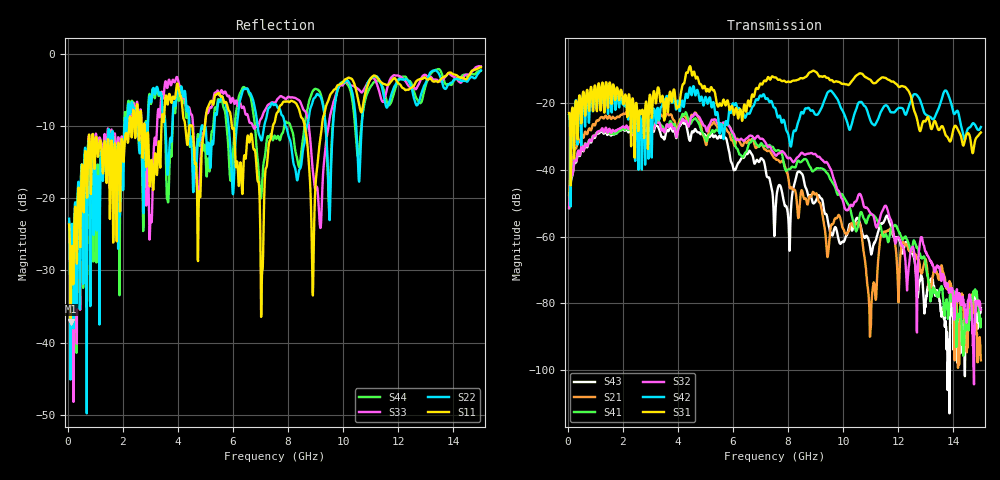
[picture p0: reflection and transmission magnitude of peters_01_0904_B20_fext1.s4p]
# MHZ S RI R 50.00
! FREQ  S11  S12  S13  S14
!  S21  S22  S23  S24
!  S31  S32  S33  S34
!  S41  S42  S43  S44
!  REAL  IMAG  REAL  IMAG  REAL  IMAG  REAL  IMAG
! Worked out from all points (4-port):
!   1496 points, 50 MHz to 15 GHz, reference 50 ohm
!   strongest paths, dB at 50 MHz, 3.79 GHz, 7.53 GHz, 11.27 GHz, 15 GHz:
!     S31: -22.9, -19.1, -12.2, -13.2, -28.8
!     S42: -23.3, -19.7, -21.4, -24.8, -27.1
!     S32: -51.3, -27.1, -35.6, -56.2, -82.0
!     S41: -50.9, -26.3, -34.2, -55.6, -84.7
!     S21: -47.5, -24.1, -36.6, -67.1, -97.1
!     S43: -51.5, -28.1, -55.1, -58.6, -81.5
!   lowest |S11| = -37.1 dB at 110 MHz (marker M1), VSWR 1.03, Z = 51.4 + j0.0826 ohm
!   |S11| at or under -10 dB: start of sweep to 2.229 GHz; 5.956 GHz to 7.451 GHz (1.495 GHz wide, 22.3 % of centre); 8.602 GHz to 9.228 GHz (625.7 MHz wide, 7.02 % of centre)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
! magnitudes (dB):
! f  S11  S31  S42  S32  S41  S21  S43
! 50 MHz  -23.7  -22.9  -23.3  -51.3  -50.9  -47.5  -51.5
! 110 MHz  -37.1  -44.7  -51.0  -43.4  -43.4  -40.1  -44.0
! 5.72 GHz  -6.7  -20.6  -26.0  -25.7  -25.9  -27.4  -30.4
! 7.05 GHz  -30.8  -14.4  -18.0  -30.7  -32.2  -32.5  -36.7
! 10.98 GHz  -3.6  -12.9  -25.0  -52.9  -53.3  -90.0  -63.5
! 11.71 GHz  -4.0  -13.3  -22.6  -54.7  -58.6  -57.6  -56.3
! 15 GHz  -1.9  -28.8  -27.1  -82.0  -84.7  -97.1  -81.5
